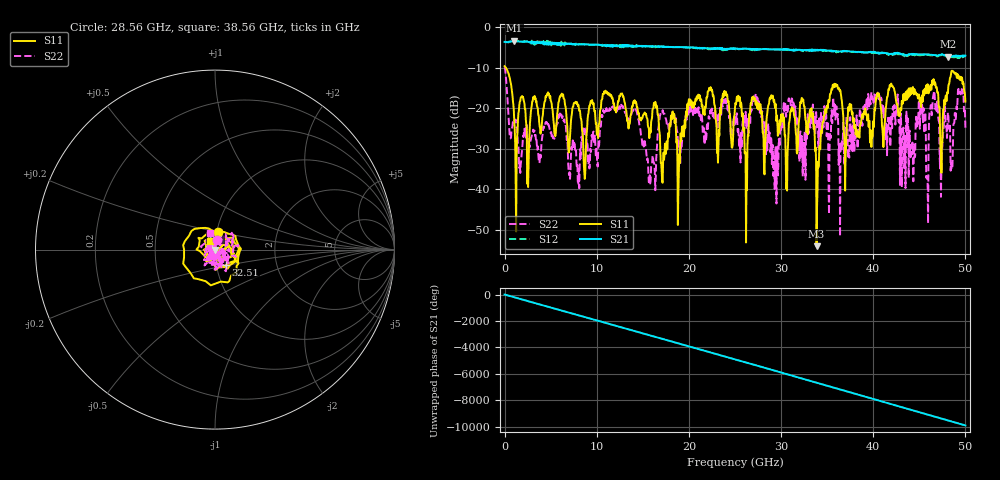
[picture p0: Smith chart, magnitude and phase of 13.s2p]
! 2/2/2024 4:24:28 PM
! D:\_XLC\ZPD9-2M1-50G-2425\13.S2P
! CHANNEL.1
! TR.MEASUREMENT
! CORRECTED.DATA
! RF.CORRECTION: FULL.TWO.PORT.CAL.PORT.1.2
! AVERAGING.OFF
! IF.BANDWIDTH: NO.IFBW
! SWEEPTYPE:  FREQ.SWEEP(Linear)
! Reference Plane Port Info
! PORT:  PORT1  PORT2
! DISTANCE:  0  m  0  m
! TIME:  0  s  0  s
! PHASE.OFFSET:  0 °  0 °
! LOSS:  0  dB  0  dB
! REF.LOSS:  0  dB  0  dB
! REF.FREQ:  0  Hz  0  Hz
! Power Info
! POWER:  0  dBm  0  dBm
! EFF.POWER:  0  dBm  0  dBm
! SOURCE.ATTEN:  0  dB  0  dB
! TEST.ATTEN:  0  dB  0  dB
# GHZ S RI R 50.0
! FREQ.GHZ  S11RE  S11IM  S21RE  S21IM  S12RE  S12IM  S22RE  S22IM
!; PortSelection: Port_12
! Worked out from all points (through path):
!   1001 points, 10 MHz to 50.01 GHz, reference 50 ohm
!   highest |S21| = -3.27 dB at 1.06 GHz (marker M1); lowest = -7.3 dB at 48.16 GHz (marker M2)
!   group delay of S21, straight-line fit = 550 ps
!   lowest |S11| = -54.1 dB at 33.86 GHz (marker M3), VSWR 1.00, Z = 50.1 - j0.136 ohm
!   |S11| at or under -10 dB: 148.4 MHz to end of sweep
!   |S22| runs from -51.7 to -9.7 dB; largest |S21 - S12| = 0.072
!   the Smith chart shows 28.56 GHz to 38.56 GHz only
!   S11 on the Smith chart (normalised r, x): 28.56 GHz: 1.02, +0.20; 32.51 GHz: 1.11, -0.19; 38.56 GHz: 0.94, +0.09
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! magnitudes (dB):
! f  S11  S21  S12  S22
! 10 MHz  -9.6  -3.6  -3.6  -9.7
! 1.06 GHz  -23.3  -3.3  -3.4  -22.8
! 8.36 GHz  -23.3  -4.2  -4.2  -27.0
! 16.71 GHz  -22.3  -4.8  -4.7  -24.9
! 25.01 GHz  -19.8  -5.3  -5.4  -22.4
! 26.21 GHz  -53.2  -5.3  -5.3  -22.1
! 26.91 GHz  -17.5  -5.5  -5.7  -17.5
! 28.56 GHz  -20.2  -5.4  -5.5  -25.6
! 29.41 GHz  -18.9  -5.5  -5.5  -29.6
! 31.06 GHz  -20.6  -5.7  -5.7  -19.3
! 32.51 GHz  -19.6  -5.6  -5.7  -34.3
! 33.36 GHz  -22.3  -5.8  -5.8  -23.7
! 33.86 GHz  -54.1  -5.7  -5.7  -23.4
! 35.71 GHz  -14.8  -5.9  -6.2  -19.1
! 38.56 GHz  -25.0  -6.1  -6.2  -20.3
! 41.71 GHz  -15.5  -6.6  -6.8  -25.2
! 45.21 GHz  -19.7  -6.7  -6.9  -21.0
! 45.81 GHz  -16.3  -6.7  -6.8  -36.9
! 46.71 GHz  -13.6  -6.9  -7.0  -18.3
! 47.41 GHz  -36.0  -6.7  -6.9  -33.9
! 48.16 GHz  -14.6  -7.3  -7.1  -21.5
! 50.01 GHz  -18.4  -7.0  -7.2  -24.9
